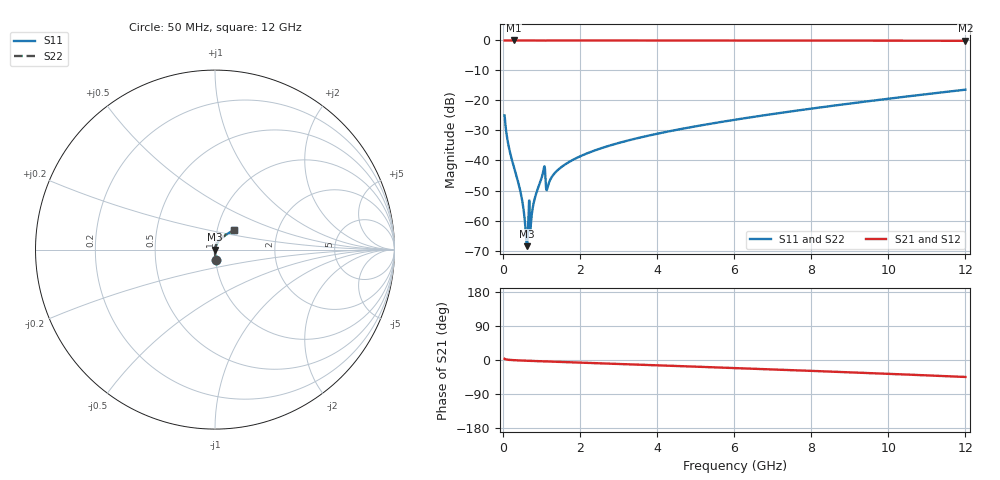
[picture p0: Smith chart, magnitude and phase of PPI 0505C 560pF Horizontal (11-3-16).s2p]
# MHz S MA R 50
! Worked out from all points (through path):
!   1601 points, 50 MHz to 12 GHz, reference 50 ohm
!   highest |S21| = 0.00 dB at 281.5 MHz (marker M1); lowest = -0.1 dB at 12 GHz (marker M2)
!   group delay of S21, straight-line fit = 10.4 ps
!   lowest |S11| = -68.5 dB at 625.1 MHz (marker M3), VSWR 1.00, Z = 50 - j0.00862 ohm
!   |S11| at or under -10 dB: start of sweep to end of sweep
!   |S22| runs from -68.5 to -16.4 dB; largest |S21 - S12| = 0
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50  0.05635 -86.8  0.9982 3.1  0.9982 3.1  0.05635 -86.8
162.0312  0.01642 -88.8  0.9996 0.4  0.9996 0.4  0.01642 -88.8
281.5312  0.008179 -88.6  0.9997 -0.4  0.9997 -0.4  0.008179 -88.6
460.7812  0.00302 -85.4  0.9997 -1.3  0.9997 -1.3  0.00302 -85.4
520.5312  0.001888 -81.7  0.9996 -1.5  0.9996 -1.5  0.001888 -81.7
587.75  0.0007875 -66.0  0.9996 -1.8  0.9996 -1.8  0.0007875 -66.0
625.0938  0.0003737 -13.3  0.9996 -1.9  0.9996 -1.9  0.0003737 -13.3
669.9062  0.001129 56.3  0.9994 -2.1  0.9994 -2.1  0.001129 56.3
722.1875  0.0007469 48.2  0.9995 -2.3  0.9995 -2.3  0.0007469 48.2
767  0.001453 71.8  0.9996 -2.5  0.9996 -2.5  0.001453 71.8
841.6875  0.002464 77.8  0.9995 -2.8  0.9995 -2.8  0.002464 77.8
1043.344  0.006184 74.5  0.9986 -3.6  0.9986 -3.6  0.006184 74.5
1177.781  0.003855 72.2  0.999 -3.9  0.999 -3.9  0.003855 72.2
1289.812  0.005513 80.0  0.9994 -4.3  0.9994 -4.3  0.005513 80.0
1446.656  0.007092 81.1  0.9994 -4.9  0.9994 -4.9  0.007092 81.1
2044.156  0.01202 80.5  0.9993 -7.0  0.9993 -7.0  0.01202 80.5
2880.656  0.01857 78.2  0.9991 -10.0  0.9991 -10.0  0.01857 78.2
4038.312  0.02818 74.6  0.9987 -14.1  0.9987 -14.1  0.02818 74.6
6025  0.04777 67.8  0.9977 -21.3  0.9977 -21.3  0.04777 67.8
8019.156  0.07337 60.6  0.9959 -28.7  0.9959 -28.7  0.07337 60.6
10013.31  0.1072 52.9  0.9926 -36.5  0.9926 -36.5  0.1072 52.9
12000  0.1512 44.8  0.9865 -44.8  0.9865 -44.8  0.1512 44.8
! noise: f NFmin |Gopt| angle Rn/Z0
50  0.0002913  0.8229  0.2174  0.0003452
1372  0.002722  0.5563  4.207  0.001098
2701  0.004143  0.4621  8.086  0.001291
4031  0.005531  0.4187  11.84  0.00154
5360  0.006844  0.3908  15.44  0.001773
6682  0.008122  0.3725  18.86  0.002002
8012  0.009408  0.3611  22.12  0.002241
9341  0.01072  0.3553  25.22  0.002499
1.067e+04  0.01209  0.3542  28.15  0.002785
1.2e+04  0.01353  0.3575  30.96  0.003109
